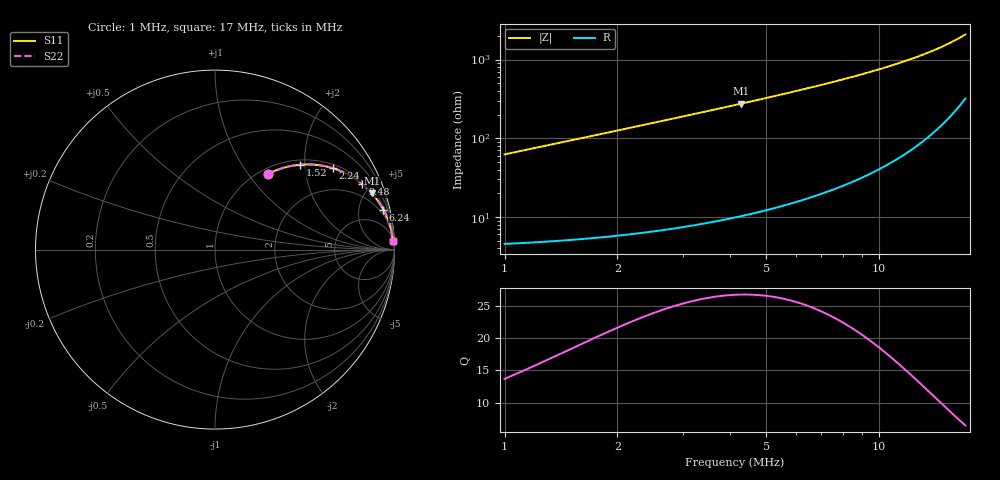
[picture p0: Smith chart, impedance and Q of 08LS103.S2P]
! Coilcraft 0805LS-103 Chip Inductor
! 18 September 2002
# MHZ S MA R 50
!Freq  MagS11  AngS11  MagS21  AngS21  MagS12  AngS12  MagS22  AngS22
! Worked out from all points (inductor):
!   401 points, 1 MHz to 17 MHz, reference 50 ohm
!   read as one part in series: L = 9.94 uH near 1.08 MHz
!   highest Q = 26.8 at 4.28 MHz (marker M1), where L = 10.2 uH
!   S11 on the Smith chart (normalised r, x): 1 MHz: 1.09, +1.25; 1.52 MHz: 1.10, +1.90; 2.24 MHz: 1.12, +2.81; 3.48 MHz: 1.17, +4.42; 6.24 MHz: 1.33, +8.32; 17 MHz: 7, +41
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1  0.5133 55.0  0.8216 -30.8  0.8216 -30.8  0.5133 55.0
1.08  0.5423 53.3  0.8038 -32.8  0.8038 -32.8  0.5423 53.3
1.28  0.6069 49.2  0.7588 -37.3  0.7588 -37.3  0.6069 49.2
1.52  0.6711 44.8  0.706 -42.1  0.706 -42.1  0.6711 44.8
1.68  0.7069 42.2  0.6724 -44.9  0.6724 -44.9  0.7069 42.2
1.88  0.745 39.2  0.6326 -48.1  0.6326 -48.1  0.745 39.2
2.24  0.7987 34.6  0.5679 -52.9  0.5679 -52.9  0.7987 34.6
2.52  0.8304 31.5  0.5237 -56.1  0.5237 -56.1  0.8304 31.5
2.8  0.8557 28.9  0.4844 -58.8  0.4844 -58.8  0.8557 28.9
3.12  0.8785 26.4  0.4448 -61.4  0.4448 -61.4  0.8785 26.4
3.48  0.8985 23.9  0.4062 -63.9  0.4062 -63.9  0.8985 23.9
3.68  0.9076 22.8  0.3871 -65.1  0.3871 -65.1  0.9076 22.8
4.28  0.9287 19.7  0.3377 -68.1  0.3377 -68.1  0.9287 19.7
5.16  0.9489 16.4  0.282 -71.5  0.282 -71.5  0.9489 16.4
6.24  0.9637 13.4  0.2316 -74.4  0.2316 -74.4  0.9637 13.4
6.36  0.965 13.1  0.2269 -74.6  0.2269 -74.6  0.965 13.1
7.6  0.9747 10.7  0.1856 -76.8  0.1856 -76.8  0.9747 10.7
9  0.9813 8.7  0.1508 -78.6  0.1508 -78.6  0.9813 8.7
11.68  0.9878 6.0  0.1041 -80.3  0.1041 -80.3  0.9878 6.0
14.36  0.9906 4.1  0.07172 -80.4  0.07172 -80.4  0.9906 4.1
15.6  0.9912 3.4  0.05965 -79.8  0.05965 -79.8  0.9912 3.4
17  0.9916 2.7  0.0476 -78.5  0.0476 -78.5  0.9916 2.7
